| Simulator:  ****** HSPICE -- O-2018.09-1 win64 (Sep 27 2018) ******
| This Model is valid for Industrial Temperature Range -40C<=Tc<=85C
| Valid for LPDDR2-1066 operation
| Part Number   VCC_N   VDD2/VDDQ   Package   Architecture
| SCP30N1G1GSL  1.8+0.15/-0.1  1.2 +0.1/-0.06  162-Ball FBGA   32Meg x 32
[IBIS ver] 5.0
[File name]  scp30n1g1gsl.ibs
[File Rev]  1.1
[Date]   2022-11-09
[Source] Simulation of a silicon level SPICE model
[Notes]  IBIS Characteristics for I/O Buffer
  IBIS Model Revision History:
  Rev 1.0:   2021-09-09 - IBIS model file initial creation
  Rev 1.1:   2022-11-09 - Add SCP30N1G1GSL
[Disclaimer]  The IBIS models are for modeling purpose only and are subject to change without any notice. UniIC is not
  responsible for any problems the models may cause.
[Copyright] Copyright 2022 UniIC Semiconductors Corp. All rights reserved
|   Component SCP30N1G1GSL
[Component] SCP30N1G1GSL
[Manufacturer] UniIC Semiconductors Corp.
[Package]
| variable   typ   min   max
R_pkg   0.542   0.214   0.99
L_pkg   2.494nH   0.885nH   4.606nH
C_pkg   0.728pF   0.371pF   1.124pF
[Pin]  signal_name   model_name   R_pin   L_pin   C_pin
|IN   dq_in   dummy
|EN   dq_en   dummy
A1	DNU1	NC	NA	NA	NA
A2	DNU2	NC	NA	NA	NA
A3	WPN	ND_CTL	0.502 	2.646nH	0.583pF
A4	CLE	ND_CTL	0.265 	1.26nH	0.372pF
A5	VCC	POWER
A6	IO4	ND_DQ	0.543 	3.069nH	0.629pF
A7	IO7	ND_DQ	0.688 	3.79nH	0.779pF
A8	VCC	POWER
A9	DNU3	NC	NA	NA	NA
A10	DNU4	NC	NA	NA	NA
B1	DNU5	NC	NA	NA	NA
B2	VCC	POWER
B3	NC1	NC	NA	NA	NA
B4	ALE	ND_CTL	0.274 	1.349nH	0.371pF
B5	REN	ND_CTL	0.295 	1.499nH	0.409pF
B6	IO5	ND_DQ	0.533 	3.025nH	0.641pF
B7	NC2	NC	NA	NA	NA
B8	NC3	NC	NA	NA	NA
B9	VSS_N	GND	NA	NA	NA
B10	DNU6	NC	NA	NA	NA
C1	NC4	NC	NA	NA	NA
C2	IO1	ND_DQ	0.718 	3.658nH	0.813pF
C3	IO3	ND_DQ	0.583 	3.224nH	0.7pF
C4	WEN	ND_CTL	0.329 	1.61nH	0.435pF
C5	RYBY	ND_RB	0.365 	2.057nH	0.479pF
C6	IO6	ND_DQ	0.508 	2.861nH	0.629pF
D1	NC5	NC	NA	NA	NA
D2	IO0	ND_DQ	0.773 	3.468nH	0.83pF
D3	IO2	ND_DQ	0.528 	3.009nH	0.641pF
D4	CEN	ND_CTL	0.269 	1.356nH	0.378pF
D5	NC6	NC	NA	NA	NA
D6	NC7	NC	NA	NA	NA
E1	VSS_N	GND	NA	NA	NA
E2	NC8	NC	NA	NA	NA
E3	NC9	NC	NA	NA	NA
E5	VDD2	POWER
E6	VDD1	POWER
E7	DQ31	DQ	0.742 	4.036nH	0.894pF
E8	DQ29	DQ	0.649 	3.718nH	0.791pF
E9	DQ26	DQ	0.615 	3.136nH	0.78pF
E10	DNU7	NC	NA	NA	NA
F1	VDD1	POWER
F2	VSS_D	GND	NA	NA	NA
F3	NC10	NC	NA	NA	NA
F5	VSS_D	GND	NA	NA	NA
F6	VSSQ	GND	NA	NA	NA
F7	VDDQ	POWER
F8	DQ25	DQ	0.661 	3.278nH	0.834pF
F9	VSSQ	GND	NA	NA	NA
F10	VDDQ	POWER
G1	VSS_D	GND	NA	NA	NA
G2	VDD2	POWER
G3	ZQ	NC	0.467 	2.29nH	0.853pF
G5	VDDQ	POWER
G6	DQ30	DQ	0.883 	4.581nH	1.038pF
G7	DQ27	DQ	0.860 	3.896nH	1.015pF
G8	DQS3_T	DQ	0.705 	3.251nH	0.889pF
G9	DQS3_C	DQ	0.665 	3.065nH	0.843pF
G10	VSSQ	GND	NA	NA	NA
H1	VSS_D	GND	NA	NA	NA
H2	CA9	CA	0.440 	2.25nH	0.771pF
H3	CA8	CA	0.428 	2.241nH	0.757pF
H5	DQ28	DQ	0.990 	4.606nH	1.124pF
H6	DQ24	DQ	0.861 	3.809nH	1.028pF
H7	DM3	DQ	0.713 	3.162nH	0.871pF
H8	DQ15	DQ	0.631 	2.933nH	0.799pF
H9	VDDQ	POWER
H10	VSSQ	GND	NA	NA	NA
J1	NC11	NC	NA	NA	NA
J2	CA6	CA	0.424 	2.258nH	0.78pF
J3	CA7	CA	0.367 	1.993nH	0.699pF
J5	VSSQ	GND	NA	NA	NA
J6	DQ11	DQ	0.723 	3.259nH	0.874pF
J7	DQ13	DQ	0.625 	3.039nH	0.802pF
J8	DQ14	DQ	0.555 	2.737nH	0.725pF
J9	DQ12	DQ	0.536 	2.617nH	0.708pF
J10	VDDQ	POWER
K1	VDD2	POWER
K2	CA5	CA	0.440 	2.275nH	0.815pF
K3	VREFCA	POWER
K5	DQS1_C	DQ	0.746 	3.5nH	0.896pF
K6	DQS1_T	DQ	0.745 	3.375nH	0.904pF
K7	DQ10	DQ	0.630 	2.996nH	0.79pF
K8	DQ9	DQ	0.538 	2.711nH	0.689pF
K9	DQ8	DQ	0.595 	2.809nH	0.768pF
K10	VSSQ	GND	NA	NA	NA
L1	NC12	NC	NA	NA	NA
L2	VSS_D	GND	NA	NA	NA
L3	CK_C	CA	0.425 	2.016nH	0.776pF
L5	DM1	DQ	0.680 	3.275nH	0.805pF
L6	VDDQ	POWER
M1	VSS_D	GND	NA	NA	NA
M2	NC13	NC	NA	NA	NA
M3	CK_T	CA	0.407 	1.818nH	0.762pF
M5	VSSQ	GND	NA	NA	NA
M6	VDDQ	POWER
M7	VDD2	POWER
M8	VSS_D	GND	NA	NA	NA
M9	VREFDQ	POWER
N1	CKE	CKE	0.517 	2.453nH	0.878pF
N2	NC14	NC	NA	NA	NA
N3	NC15	NC	NA	NA	NA
N5	DM0	DQ	0.670 	3.153nH	0.793pF
N6	VDDQ	POWER
P1	CS_N	CA	0.447 	2.366nH	0.774pF
P2	NC16	NC	NA	NA	NA
P3	NC17	NC	NA	NA	NA
P5	DQS0_C	DQ	0.714 	3.216nH	0.867pF
P6	DQS0_T	DQ	0.714 	2.963nH	0.882pF
P7	DQ5	DQ	0.515 	2.307nH	0.675pF
P8	DQ6	DQ	0.495 	2.255nH	0.664pF
P9	DQ7	DQ	0.436 	1.881nH	0.607pF
P10	VSSQ	GND	NA	NA	NA
R1	CA4	CA	0.387 	1.896nH	0.741pF
R2	CA3	CA	0.281 	1.26nH	0.603pF
R3	CA2	CA	0.331 	1.362nH	0.65pF
R5	VSSQ	GND	NA	NA	NA
R6	DQ4	DQ	0.626 	2.501nH	0.789pF
R7	DQ2	DQ	0.561 	2.3nH	0.724pF
R8	DQ1	DQ	0.491 	2.06nH	0.648pF
R9	DQ3	DQ	0.437 	1.867nH	0.611pF
R10	VDDQ	POWER
T1	VSS_D	GND	NA	NA	NA
T2	NC18	NC	NA	NA	NA
T3	CA1	CA	0.245 	1.003nH	0.597pF
T5	DQ19	DQ	0.708 	3.038nH	0.853pF
T6	DQ23	DQ	0.660 	2.694nH	0.814pF
T7	DM2	DQ	0.506 	2.101nH	0.663pF
T8	DQ0	DQ	0.484 	2.119nH	0.628pF
T9	VDDQ	POWER
T10	VSSQ	GND	NA	NA	NA
U1	VSS_D	GND	NA	NA	NA
U2	VDD2	POWER
U3	CA0	CA	0.214 	0.885nH	0.577pF
U5	VDDQ	POWER
U6	DQ17	DQ	0.596 	2.783nH	0.754pF
U7	DQ20	DQ	0.588 	2.421nH	0.752pF
U8	DQS2_T	DQ	0.430 	1.885nH	0.595pF
U9	DQS2_C	DQ	0.403 	1.743nH	0.577pF
U10	VSSQ	GND	NA	NA	NA
V1	VDD1	POWER
V2	VSS_D	GND	NA	NA	NA
V3	NC19	NC	NA	NA	NA
V5	VSS_D	GND	NA	NA	NA
V6	VSSQ	GND	NA	NA	NA
V7	VDDQ	POWER
V8	DQ22	DQ	0.443 	2.004nH	0.618pF
V9	VSSQ	GND	NA	NA	NA
V10	VDDQ	POWER
W1	DNU8	NC	NA	NA	NA
W2	NC20	NC	NA	NA	NA
W3	NC21	NC	NA	NA	NA
W5	VDD2	POWER
W6	VDD1	POWER
W7	DQ16	DQ	0.534 	2.438nH	0.665pF
W8	DQ18	DQ	0.433 	2.125nH	0.587pF
W9	DQ21	DQ	0.334 	1.493nH	0.503pF
W10	DNU9	NC	NA	NA	NA
Y1	DNU10	NC	NA	NA	NA
Y2	DNU11	NC	NA	NA	NA
Y9	DNU12	NC	NA	NA	NA
Y10	DNU13	NC	NA	NA	NA
|***********************PIN MAPPING*****************************************
[Pin Mapping]	pulldown_ref	pullup_ref	gnd_clamp_ref	power_clamp_ref ext_ref
A1	NC	NC
A2	NC	NC
A3   VSS_N	VCC_N	VSS_N	VCC_N
A4	VSS_N	VCC_N	VSS_N	VCC_N
A5	NC	VCC_N
A6	VSS_N	VCC_N	VSS_N	VCC_N
A7	VSS_N	VCC_N	VSS_N	VCC_N
A8	NC	VCC_N
A9	NC	NC
A10	NC	NC
B1	NC	NC
B2	NC	VCC_N
B3	NC	NC
B4	VSS_N	VCC_N	VSS_N	VCC_N
B5	VSS_N	VCC_N	VSS_N	VCC_N
B6	VSS_N	VCC_N	VSS_N	VCC_N
B7	NC	NC
B8	NC	NC
B9	VSS_N	NC
B10	NC	NC
C1	NC	NC
C2	VSS_N	VCC_N	VSS_N	VCC_N
C3	VSS_N	VCC_N	VSS_N	VCC_N
C4	VSS_N	VCC_N	VSS_N	VCC_N
C5	VSS_N	VCC_N	VSS_N	VCC_N
C6	VSS_N	VCC_N	VSS_N	VCC_N
D1	NC	NC
D2	VSS_N	VCC_N	VSS_N	VCC_N
D3	VSS_N	VCC_N	VSS_N	VCC_N
D4	VSS_N	VCC_N	VSS_N	VCC_N
D5	NC	NC
D6	NC	NC
E1	VSS_N	NC
E2	NC	NC
E3	NC	NC
E5	NC	VDD2
E6	NC	VDD1
E7	VSSQ	VDDQ	VSSQ	VDDQ
E8	VSSQ	VDDQ	VSSQ	VDDQ
E9	VSSQ	VDDQ	VSSQ	VDDQ
E10	NC	NC
F1	NC	VDD1
F2	VSS_D	NC
F3	NC	NC
F5	VSS_D	NC
F6	VSSQ	NC
F7	NC	VDDQ
F8	VSSQ	VDDQ	VSSQ	VDDQ
F9	VSSQ	NC
F10	NC	VDDQ
G1	VSS_D	NC
G2	NC	VDD2
G3	NC	NC
G5	NC	VDDQ
G6	VSSQ	VDDQ	VSSQ	VDDQ
G7	VSSQ	VDDQ	VSSQ	VDDQ
G8	VSSQ	VDDQ	VSSQ	VDDQ
G9	VSSQ	VDDQ	VSSQ	VDDQ
G10	VSSQ	NC
H1	VSS_D	NC
H2	VSS_D	VDD2	VSS_D	VDD2
H3	VSS_D	VDD2	VSS_D	VDD2
H5	VSSQ	VDDQ	VSSQ	VDDQ
H6	VSSQ	VDDQ	VSSQ	VDDQ
H7	VSSQ	VDDQ	VSSQ	VDDQ
H8	VSSQ	VDDQ	VSSQ	VDDQ
H9	NC	VDDQ
H10	VSSQ	NC
J1	NC	NC
J2	VSS_D	VDD2	VSS_D	VDD2
J3	VSS_D	VDD2	VSS_D	VDD2
J5	VSSQ	NC
J6	VSSQ	VDDQ	VSSQ	VDDQ
J7	VSSQ	VDDQ	VSSQ	VDDQ
J8	VSSQ	VDDQ	VSSQ	VDDQ
J9	VSSQ	VDDQ	VSSQ	VDDQ
J10	NC	VDDQ
K1	NC	VDD2
K2	VSS_D	VDD2	VSS_D	VDD2
K3	NC  	VREFCA
K5	VSSQ	VDDQ	VSSQ	VDDQ
K6	VSSQ	VDDQ	VSSQ	VDDQ
K7	VSSQ	VDDQ	VSSQ	VDDQ
K8	VSSQ	VDDQ	VSSQ	VDDQ
K9	VSSQ	VDDQ	VSSQ	VDDQ
K10	VSSQ	NC
L1	NC	NC
L2	VSS_D	NC
L3	VSS_D	VDD2	VSS_D	VDD2
L5	VSSQ	VDDQ	VSSQ	VDDQ
L6	NC	VDDQ
M1	VSS_D	NC
M2	NC	NC
M3	VSS_D	VDD2	VSS_D	VDD2
M5	VSSQ	NC
M6	NC	VDDQ
M7	NC	VDD2
M8	VSS_D	NC
M9	NC 	VREFDQ
N1	VSS_D	VDD2	VSS_D	VDD2
N2	NC	NC
N3	NC	NC
N5	VSSQ	VDDQ	VSSQ	VDDQ
N6	NC	VDDQ
P1	VSS_D	VDD2	VSS_D	VDD2
P2	NC	NC
P3	NC	NC
P5	VSSQ	VDDQ	VSSQ	VDDQ
P6	VSSQ	VDDQ	VSSQ	VDDQ
P7	VSSQ	VDDQ	VSSQ	VDDQ
P8	VSSQ	VDDQ	VSSQ	VDDQ
P9	VSSQ	VDDQ	VSSQ	VDDQ
P10	VSSQ	NC
R1	VSS_D	VDD2	VSS_D	VDD2
R2	VSS_D	VDD2	VSS_D	VDD2
R3	VSS_D	VDD2	VSS_D	VDD2
R5	VSSQ	NC
R6	VSSQ	VDDQ	VSSQ	VDDQ
R7	VSSQ	VDDQ	VSSQ	VDDQ
R8	VSSQ	VDDQ	VSSQ	VDDQ
R9	VSSQ	VDDQ	VSSQ	VDDQ
R10	NC	VDDQ
T1	VSS_D	NC
T2	NC	NC
T3	VSS_D	VDD2	VSS_D	VDD2
T5	VSSQ	VDDQ	VSSQ	VDDQ
T6	VSSQ	VDDQ	VSSQ	VDDQ
T7	VSSQ	VDDQ	VSSQ	VDDQ
T8	VSSQ	VDDQ	VSSQ	VDDQ
T9	NC	VDDQ
T10	VSSQ	NC
U1	VSS_D	NC
U2	NC	VDD2
U3	VSS_D	VDD2	VSS_D	VDD2
U5	NC	VDDQ
U6	VSSQ	VDDQ	VSSQ	VDDQ
U7	VSSQ	VDDQ	VSSQ	VDDQ
U8	VSSQ	VDDQ	VSSQ	VDDQ
U9	VSSQ	VDDQ	VSSQ	VDDQ
U10	VSSQ	NC
V1	NC	VDD1
V2	VSS_D	NC
V3	NC	NC
V5	VSS_D	NC
V6	VSSQ	NC
V7	NC	VDDQ
V8	VSSQ	VDDQ	VSSQ	VDDQ
V9	VSSQ	NC
V10	NC	VDDQ
W1	NC	NC
W2	NC	NC
W3	NC	NC
W5	NC	VDD2
W6	NC	VDD1
W7	VSSQ	VDDQ	VSSQ	VDDQ
W8	VSSQ	VDDQ	VSSQ	VDDQ
W9	VSSQ	VDDQ	VSSQ	VDDQ
W10	NC	NC
Y1	NC	NC
Y2	NC	NC
Y9	NC	NC
Y10	NC	NC
[Diff pin]  inv_pin  vdiff   tdelay_typ   tdelay_min   tdelay_max
H3   L3   0.300V   NA   NA   NA
P6   P5   0.300V   NA   NA   NA
K6   K5   0.300V   NA   NA   NA
U8   U9   0.300V   NA   NA   NA
G8   G9   0.300V   NA   NA   NA
[Model Selector] DQ
DQ_RON240  RON=240ohms
DQ_RON120  RON=120ohms
DQ_RON80  RON=80ohms
DQ_RON60  RON=60ohms
DQ_RON48  RON=48ohms
DQ_RON40  RON=40ohms
DQ_RON34  RON=34ohms
DQ_RCV_ODTOFF  DQ_RCV_ODTOFF&LPDDR2 Default
DQ_RCV_ODT240  DQ_RCV_ODT240
DQ_RCV_ODT120  DQ_RCV_ODT120
DQ_RCV_ODT60  DQ_RCV_ODT60
| Models and submodels in the file (19): DQ_RON240 (I/O), DQ_RON120 (I/O), DQ_RON80 (I/O), DQ_RON60 (I/O), DQ_RON48 (I/O), DQ_RON40 (I/O), DQ_RON34 (I/O), DQ_RCV_ODTOFF (Input), DQ_RCV_ODT240 (Input), DQ_RCV_ODT120 (Input), DQ_RCV_ODT60 (Input), CA (Input), CKE (Input), ND_CTL (Input), ND_DQ (I/O), ND_RB (Open_drain), DQ_ODT240 (Dynamic_clamp), DQ_ODT120 (Dynamic_clamp), DQ_ODT60 (Dynamic_clamp)
